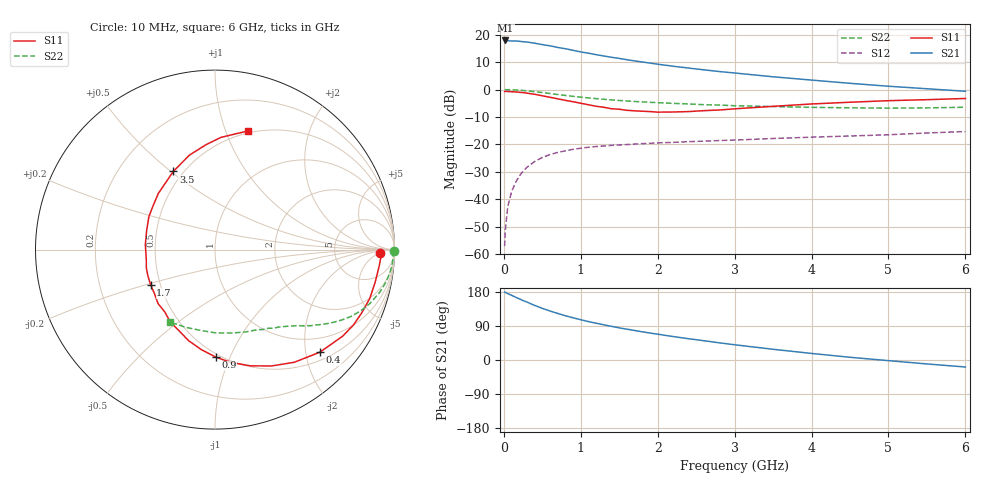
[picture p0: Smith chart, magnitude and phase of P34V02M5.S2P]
! SIEMENS Small Signal Semiconductors
! BFP181
! Si NPN RF Bipolar Junction Transistor in SOT143
! VCE = 4 V  IC = 2.5 mA
! Common Emitter S-Parameters:  March  1996
# GHz  S  MA  R  50
!  f  S11  S21  S12  S22
! GHz  MAG  ANG  MAG  ANG  MAG  ANG  MAG  ANG
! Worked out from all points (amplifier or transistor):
!   36 points, 10 MHz to 6 GHz, reference 50 ohm
!   highest |S21| = 17.9 dB at 20 MHz (marker M1)
!   |S21| within 3 dB of that: start of sweep to 797.6 MHz
!   unconditionally stable (mu >= 1): 2.295 GHz to end of sweep
!   at 250 MHz: K = 0.14, MSG = 23.6 dB, |S12| = -29.8 dB
!   at 1.4 GHz: K = 0.70, MSG = 16.0 dB, |S12| = -20.4 dB
!   at 6 GHz: K = 1.12, MAG = 5.3 dB, |S12| = -15.3 dB
!   S11 on the Smith chart (normalised r, x): 10 MHz: 23, -6; 400 MHz: 0.67, -2.29; 900 MHz: 0.47, -0.89; 1.7 GHz: 0.44, -0.21; 3.5 GHz: 0.44, +0.51; 6 GHz: 0.48, +1.20
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0.01  0.921 -1.2  7.766 179.1  0.0014 78.5  0.9954 -0.5
0.02  0.9253 -2.6  7.824 178.5  0.0028 87.4  0.993 -0.9
0.05  0.9197 -5.6  7.76 175.3  0.0072 90.4  0.993 -2.6
0.1  0.9108 -11.5  7.64 170.8  0.0137 82.0  0.9901 -5.2
0.15  0.9042 -17.5  7.658 166.0  0.0199 80.2  0.9819 -7.8
0.25  0.8783 -28.6  7.422 156.8  0.0324 73.2  0.9593 -12.6
0.3  0.8591 -34.2  7.339 153.0  0.0382 70.0  0.9456 -14.9
0.4  0.8177 -44.3  6.976 144.1  0.0487 64.1  0.9136 -19.2
0.5  0.768 -54.8  6.573 136.3  0.0579 59.0  0.8807 -22.8
0.6  0.7211 -64.0  6.261 129.3  0.0653 54.3  0.8452 -26.1
0.8  0.6345 -82.0  5.532 116.7  0.0763 46.8  0.7793 -31.2
0.9  0.599 -89.6  5.173 111.4  0.0814 43.8  0.7503 -33.3
1.1  0.528 -106.2  4.588 101.3  0.0887 38.9  0.7024 -36.7
1.4  0.4459 -128.8  3.865 88.8  0.096 33.7  0.6471 -41.1
1.7  0.4087 -151.2  3.315 77.9  0.1014 30.1  0.6053 -44.7
1.9  0.3961 -164.9  3.027 71.2  0.1047 28.2  0.5847 -47.0
2.2  0.3892 175.7  2.655 61.9  0.1089 26.5  0.5582 -50.7
2.8  0.4234 144.3  2.125 45.3  0.1176 23.2  0.5202 -58.9
3.5  0.4935 118.1  1.704 28.3  0.1281 20.7  0.4893 -69.7
4.5  0.5862 95.0  1.296 7.2  0.1422 16.6  0.4641 -89.4
5.5  0.6526 80.4  1.032 -10.4  0.1614 14.0  0.4628 -110.7
6  0.6864 74.4  0.929 -18.5  0.1716 11.5  0.4751 -121.7
